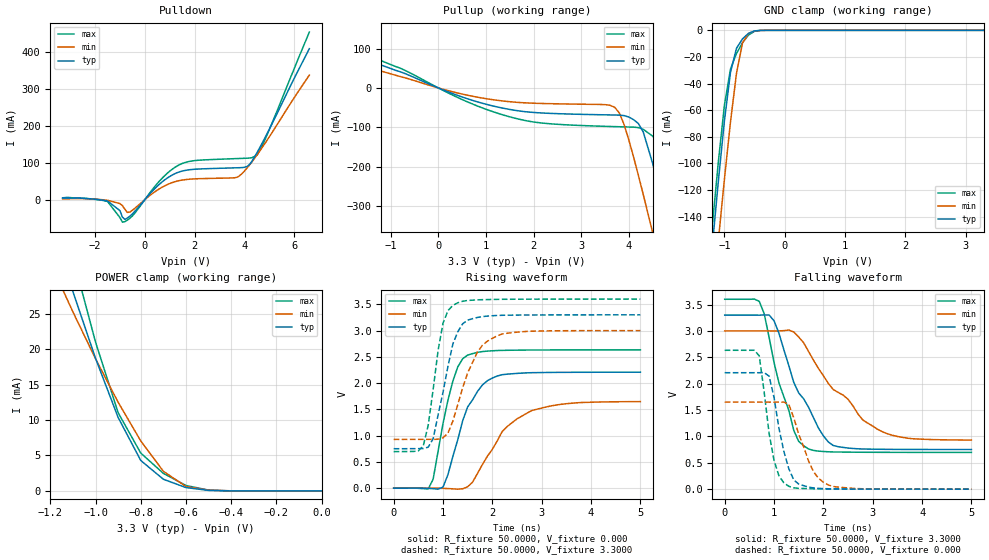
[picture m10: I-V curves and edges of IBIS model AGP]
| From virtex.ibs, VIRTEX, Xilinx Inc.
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|   Model AGP
[Model]   AGP
Model_type   I/O
Polarity   Non-Inverting
Enable   Active-Low
Vinl =   1.120V
Vinh =   1.520V
| Vmeas depends on rising or falling edge, select one of the following:
| For rising edge:
|Vmeas =   0.940V
| For falling edge:
|Vmeas =   2.00V
Cref =  10.0000pF
Rref =  50.0000
| Vref depends on rising or falling edge, select one of the following:
| For rising edge:
|Vref =   0.00V
| For falling edge:
|Vref =   3.30V
C_comp   6.5000pF   5.0000pF   8.0000pF
[Temperature Range]   27.0000   100.0000   0.000
[Voltage Range]   3.3000V   3.0000V   3.6000V
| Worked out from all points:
|   slope of the pulldown table from 0 to 0.495 V, typ, clamps not added: 13.7 ohm
|   slope of the pullup table from 0 to 0.495 V, typ, clamps not added: 21.7 ohm
|   GND clamp passes 1 mA (typ) near -0.53 V on its own axis
|   POWER clamp passes 1 mA (typ) near -0.64 V on its own axis
|   rising waveform, R_fixture 50.0000, V_fixture 0.000: 20-80 % time 499ps typ, 771ps min, 358ps max; typ from 0 V to 2.21 V
|   rising waveform, R_fixture 50.0000, V_fixture 3.3000: 20-80 % time 348ps typ, 473ps min, 265ps max; typ from 0.751 V to 3.3 V
|   falling waveform, R_fixture 50.0000, V_fixture 3.3000: 20-80 % time 695ps typ, 1.06ns min, 488ps max; typ from 3.3 V to 0.752 V
|   falling waveform, R_fixture 50.0000, V_fixture 0.000: 20-80 % time 290ps typ, 392ps min, 245ps max; typ from 2.21 V to 0 V
[Pulldown]
| voltage   I(typ)   I(min)   I(max)
-3.3V     4mA        2mA        5mA
-1.5V     -3.6mA     -1.8mA     -4.9mA
-1V       -29.72mA   -10.6mA    -48.43mA
-900mV    -47.38mA   -16.34mA   -60.95mA
-600mV    -44.69mA   -33.47mA   -50.35mA
600mV     42.54mA    29.94mA    51.16mA
1.4V      75.27mA    51.64mA    94.7mA
3.7V      86.04mA    60.44mA    110.9mA
4.1V      89.49mA    85.22mA    111.9mA
4.5V      126.6mA    120.5mA    120.3mA
4.9V      177.6mA    159.9mA    174.2mA
6.6V      407.8mA    336.3mA    452.6mA
[Pullup]
| voltage   I(typ)   I(min)   I(max)
-3.3V     137.4mA    116.7mA    152.3mA
-1.5V     71.46mA    53.37mA    84.23mA
1.4V      -52.42mA   -33.71mA   -70.06mA
3.6V      -68.53mA   -44mA      -97.91mA
3.8V      -69.08mA   -63.63mA   -98.58mA
4.2V      -90.62mA   -222.7mA   -100.8mA
4.3V      -111.5mA   -270.4mA   -105mA
4.5V      -192.3mA   -368.3mA   -122.6mA
4.7V      -290.4mA   -468.2mA   -157.6mA
4.9V      -393.7mA   -569.2mA   -241mA
5.1V      -499.3mA   -670.9mA   -340.5mA
6.6V      -1.31A     -1.442A    -1.157A
[GND_clamp]
| voltage   I(typ)   I(min)   I(max)
-3.3V     -1.286A    -1.272A    -1.289A
-1.2V     -161.8mA   -205.3mA   -146.7mA
-1.1V     -113.2mA   -157.8mA   -98.56mA
-1V       -68.04mA   -112mA     -56.27mA
-900mV    -31.6mA    -69.09mA   -29.2mA
-800mV    -13.5mA    -32.34mA   -17.42mA
-700mV    -6.408mA   -9.455mA   -9.303mA
-600mV    -2.237mA   -2.349mA   -3.538mA
-500mV    -423.5uA   -545.3uA   -698.2uA
-400mV    -42.44uA   -91.25uA   -59.93uA
3.3V      523.9pA    1.466uA    349.2pA
[POWER_clamp]
| voltage   I(typ)   I(min)   I(max)
-3.3V     276.4mA    201.2mA    346.2mA
-1.2V     38.21mA    32.25mA    46.01mA
-1.1V     28.13mA    25.27mA    33mA
-1V       18.72mA    18.66mA    21.02mA
-900mV    10.37mA    12.52mA    11.04mA
-800mV    4.3mA      7.057mA    5.343mA
-700mV    1.647mA    2.774mA    2.48mA
-600mV    473.1uA    621.1uA    767.7uA
-500mV    71.72uA    106uA      114.9uA
-400mV    5.959uA    14.29uA    7.91uA
0V        523.9pA    8.324nA    407.5pA
[Ramp]
| variable   typ   min   max
dV/dt_r   1.3242/0.4971n   0.9888/0.7709n   1.5792/0.3468n
dV/dt_f   1.5287/0.6912n   1.2413/1.0958n   1.7416/0.4938n
R_load = 50.0000
[Rising Waveform]
R_fixture = 50.0000
V_fixture = 0.000
| time   V(typ)   V(min)   V(max)
0s        0V         0V         0V
700ps     -3.8mV     862.5uV    -14.13mV
800ps     -9.51mV    982.4uV    170.4mV
1ns       21.17mV    -3.713mV   1.232V
1.3ns     925mV      -18.54mV   2.309V
1.5ns     1.547V     27.03mV    2.533V
2ns       2.096V     739.6mV    2.615V
2.3ns     2.17V      1.172V     2.624V
2.8ns     2.198V     1.478V     2.629V
5ns       2.207V     1.648V     2.632V
[Rising Waveform]
R_fixture = 50.0000
V_fixture = 3.3000
V_fixture_min = 3.0000
V_fixture_max = 3.6000
| time   V(typ)   V(min)   V(max)
0s        751.2mV    928.2mV    696.8mV
600ps     755.2mV    928.8mV    804.3mV
700ps     780.4mV    929mV      1.195V
800ps     939.8mV    928.5mV    1.876V
1ns       1.823V     959.2mV    3.139V
1.2ns     2.746V     1.276V     3.479V
1.4ns     3.13V      1.916V     3.558V
1.7ns     3.25V      2.596V     3.584V
2.1ns     3.287V     2.901V     3.593V
5ns       3.299V     2.999V     3.599V
[Falling Waveform]
R_fixture = 50.0000
V_fixture = 3.3000
V_fixture_min = 3.0000
V_fixture_max = 3.6000
| time   V(typ)   V(min)   V(max)
0s        3.3V       3V         3.6V
700ps     3.299V     3V         3.562V
800ps     3.303V     3V         3.33V
1ns       3.192V     2.999V     2.401V
1.4ns     2.024V     2.98V      1.114V
1.7ns     1.552V     2.61V      761.6mV
2ns       1.011V     2.151V     714.3mV
2.2ns     828.1mV    1.89V      706mV
3.1ns     757.3mV    1.134V     699.1mV
5ns       752.1mV    931.2mV    697.4mV
[Falling Waveform]
R_fixture = 50.0000
V_fixture = 0.000
| time   V(typ)   V(min)   V(max)
0s        2.208V     1.651V     2.633V
700ps     2.208V     1.651V     2.529V
900ps     2.143V     1.65V      1.058V
1ns       1.738V     1.651V     545.8mV
1.1ns     1.153V     1.651V     251.5mV
1.3ns     385.2mV    1.607V     54.49mV
1.5ns     96.57mV    1.042V     16.26mV
1.8ns     23.66mV    334.1mV    8.044mV
2.1ns     8.124mV    79.81mV    4.419mV
5ns       448.4uV    515.5uV    436.4uV
